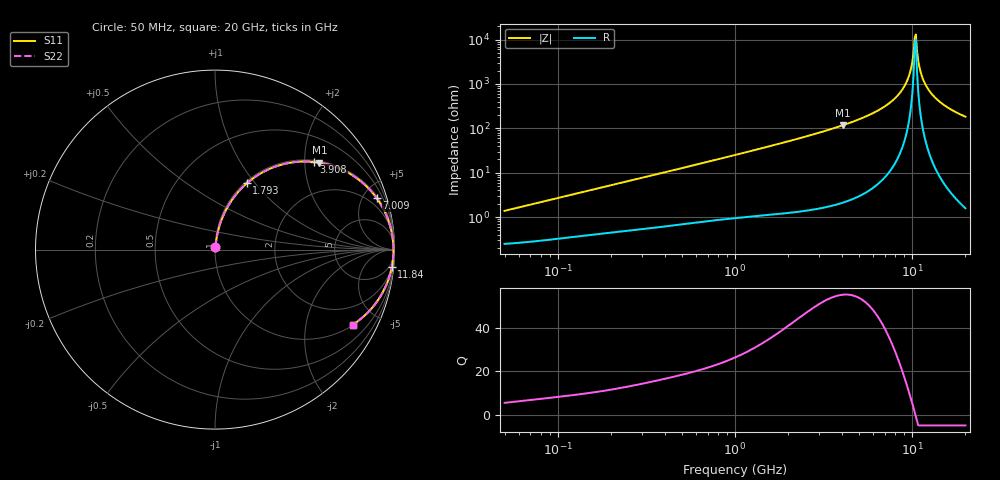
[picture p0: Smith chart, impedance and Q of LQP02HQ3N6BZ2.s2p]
!Murata Part Number: LQP02HQ3N6BZ2
!These Parameters are Measured in Series Mode Connection
!  o--[Z]--o
!Port1  Port2
!  o-------o
!Freq. Start=50[MHz] Stop=20[GHz], 401[Steps]
# Hz S RI R 50
!Freq.(Hz) S11(Real) S11(Imag) S21(Real) S21(Imag) S12(Real) S12(Imag) S22(Real) S22(Imag)
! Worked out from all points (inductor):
!   401 points, 50 MHz to 20 GHz, reference 50 ohm
!   read as one part in series: L = 4.3 nH near 51.52 MHz
!   highest Q = 55.6 at 4.088 GHz (marker M1), where L = 4.6 nH
!   self-resonance near 10.35 GHz
!   S11 on the Smith chart (normalised r, x): 50 MHz: 1.00, +0.03; 1.793 GHz: 1.02, +0.91; 3.908 GHz: 1.04, +2.23; 7.009 GHz: 1.16, +6.25; 11.84 GHz: 2, -20; 20 GHz: 1.03, -3.66
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5e7  0.00266 0.0135  0.9973 -0.0135  0.9973 -0.0135  0.00266 0.0135
1.364002e8  0.00501 0.0356  0.995 -0.0356  0.995 -0.0356  0.00501 0.0356
3.721004e8  0.0146 0.0927  0.9854 -0.0927  0.9854 -0.0927  0.0146 0.0927
1e9  0.0667 0.2314  0.9333 -0.2314  0.9333 -0.2314  0.0667 0.2314
1.793498e9  0.1777 0.3694  0.8223 -0.3694  0.8223 -0.3694  0.1777 0.3694
2.728004e9  0.3433 0.4648  0.6567 -0.4648  0.6567 -0.4648  0.3433 0.4648
3.908127e9  0.5526 0.4883  0.4474 -0.4883  0.4474 -0.4883  0.5526 0.4883
4.087748e9  0.5817 0.4844  0.4183 -0.4844  0.4183 -0.4844  0.5817 0.4844
5.515528e9  0.7738 0.4088  0.2262 -0.4088  0.2262 -0.4088  0.7738 0.4088
7.009217e9  0.9012 0.2861  0.0988 -0.2861  0.0988 -0.2861  0.9012 0.2861
7.442007e9  0.926 0.2481  0.074 -0.2481  0.074 -0.2481  0.926 0.2481
8.516016e9  0.9686 0.1543  0.0314 -0.1543  0.0314 -0.1543  0.9686 0.1543
9.316812e9  0.9859 0.0874  0.0141 -0.0874  0.0141 -0.0874  0.9859 0.0874
9.745021e9  0.991 0.053  0.009 -0.053  0.009 -0.053  0.991 0.053
1.019291e10  0.9937 0.0184  0.00633 -0.0184  0.00633 -0.0184  0.9937 0.0184
1.034674e10  0.994 0.00681  0.00599 -0.00681  0.00599 -0.00681  0.994 0.00681
1.066139e10  0.9939 -0.0164  0.00611 0.0164  0.00611 0.0164  0.9939 -0.0164
1.115139e10  0.9917 -0.0511  0.00833 0.0511  0.00833 0.0511  0.9917 -0.0511
1.183995e10  0.9849 -0.0969  0.0151 0.0969  0.0151 0.0969  0.9849 -0.0969
1.276073e10  0.9706 -0.1529  0.0294 0.1529  0.0294 0.1529  0.9706 -0.1529
1.438523e10  0.9345 -0.2375  0.0655 0.2375  0.0655 0.2375  0.9345 -0.2375
2e10  0.7685 -0.4175  0.2315 0.4175  0.2315 0.4175  0.7685 -0.4175
